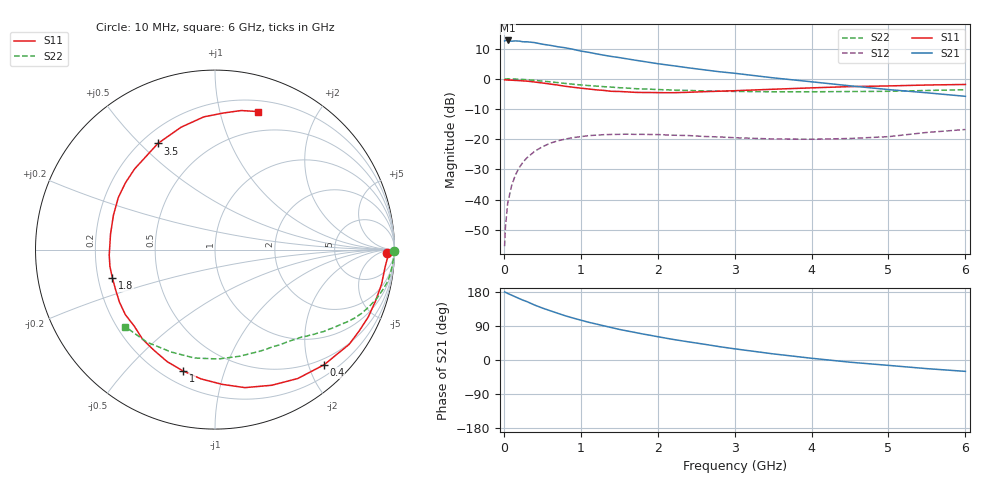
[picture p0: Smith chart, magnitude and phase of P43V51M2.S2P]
! SIEMENS Small Signal Semiconductors
! BFP182
! Si NPN RF Bipolar Junction Transistor in SOT143
! VCE = 3.5 V  IC = 1.2 mA
! Common Emitter S-Parameters:  March  1996
# GHz  S  MA  R  50
!  f  S11  S21  S12  S22
! GHz  MAG  ANG  MAG  ANG  MAG  ANG  MAG  ANG
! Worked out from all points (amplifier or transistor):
!   36 points, 10 MHz to 6 GHz, reference 50 ohm
!   highest |S21| = 12.7 dB at 50 MHz (marker M1)
!   |S21| within 3 dB of that: start of sweep to 912.6 MHz
!   unconditionally stable (mu >= 1): 2.54 GHz to end of sweep
!   at 250 MHz: K = 0.10, MSG = 19.9 dB, |S12| = -27.6 dB
!   at 1.4 GHz: K = 0.57, MSG = 12.9 dB, |S12| = -18.4 dB
!   at 6 GHz: K = 1.05, MAG = 4.2 dB, |S12| = -16.8 dB
!   S11 on the Smith chart (normalised r, x): 10 MHz: 39, -18; 400 MHz: 0.39, -2.27; 1 GHz: 0.28, -0.73; 1.8 GHz: 0.26, -0.13; 3.5 GHz: 0.26, +0.57; 6 GHz: 0.30, +1.31
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0.01  0.9588 -1.1  4.212 179.5  0.0017 91.7  0.9977 -0.4
0.02  0.9633 -2.4  4.305 178.8  0.0034 90.3  0.9913 -0.9
0.05  0.9524 -6.0  4.307 175.6  0.0087 88.9  0.9968 -2.2
0.1  0.9478 -11.8  4.19 171.2  0.0169 81.2  0.9925 -4.4
0.15  0.939 -17.8  4.236 166.7  0.0255 79.0  0.9884 -6.7
0.2  0.9328 -23.7  4.2 162.1  0.0339 75.7  0.983 -8.9
0.25  0.9224 -29.4  4.093 157.8  0.0419 72.2  0.975 -11.0
0.3  0.9152 -35.2  4.091 154.1  0.0492 68.8  0.9646 -12.9
0.4  0.8837 -46.6  3.969 145.0  0.063 62.1  0.9417 -16.8
0.6  0.8193 -67.3  3.58 130.2  0.0857 50.1  0.8907 -23.5
0.7  0.7871 -77.7  3.393 123.3  0.094 45.0  0.8647 -26.3
0.8  0.7516 -87.0  3.254 116.6  0.1007 40.5  0.8376 -28.8
1  0.6994 -104.7  2.875 105.2  0.1103 31.9  0.7914 -33.3
1.1  0.6788 -113.1  2.747 99.7  0.1146 28.5  0.7728 -35.2
1.5  0.6172 -144.1  2.244 80.8  0.1204 17.2  0.712 -42.0
1.8  0.5932 -164.5  1.949 68.9  0.1205 11.5  0.6793 -46.4
2.2  0.5884 171.6  1.645 54.3  0.1166 5.8  0.651 -52.6
2.8  0.6226 143.2  1.309 35.3  0.109 1.7  0.6241 -62.8
3.5  0.6714 118.3  1.037 16.2  0.101 2.8  0.61 -76.8
4.5  0.7422 94.8  0.765 -5.8  0.1028 10.4  0.6148 -100.8
5.5  0.7885 79.3  0.586 -22.8  0.1295 16.9  0.6406 -126.6
6  0.8055 72.7  0.513 -30.0  0.1448 15.2  0.6589 -139.3
